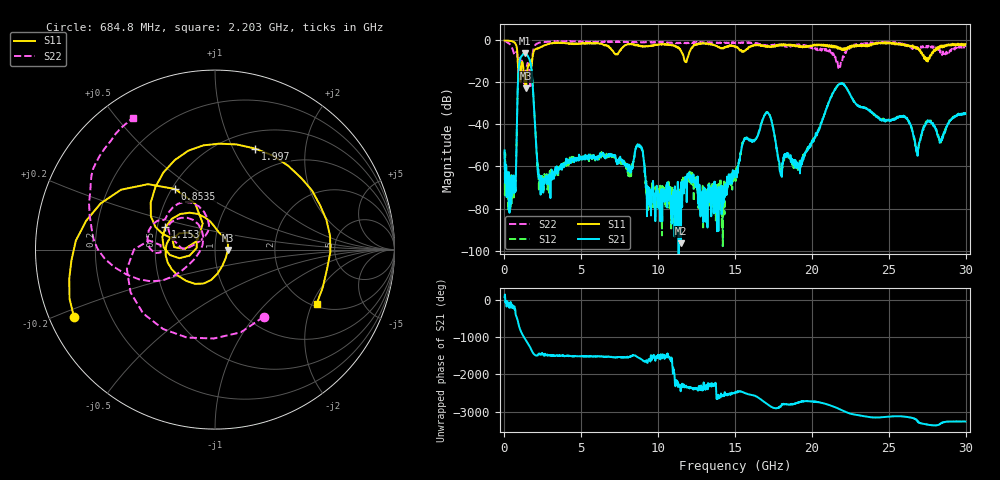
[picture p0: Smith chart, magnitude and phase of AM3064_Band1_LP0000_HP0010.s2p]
# Hz S DB R 50.0
!freq dBS11 angS11 dBS21 angS21 dBS12 angS12 dBS22 angS22
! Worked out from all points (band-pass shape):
!   1600 points, 10 MHz to 29.98 GHz, reference 50 ohm
!   highest |S21| = -6.23 dB at 1.322 GHz (marker M1); lowest = -96.5 dB at 11.48 GHz (marker M2)
!   |S21| within 3 dB of the highest: 1.008 GHz to 1.641 GHz (632.8 MHz wide, 47.8 % of centre)
!   lowest |S11| = -22.9 dB at 1.397 GHz (marker M3), VSWR 1.16, Z = 57.7 - j0.151 ohm
!   |S11| at or under -10 dB: 865.7 MHz to 1.796 GHz (930 MHz wide, 69.9 % of centre); 11.74 GHz to 11.85 GHz (101.1 MHz wide, 0.857 % of centre); 27.53057 GHz to 27.5447 GHz (14.13 MHz wide, 0.0513 % of centre)
!   |S22| runs from -22.7 to -0.2 dB; largest |S21 - S12| = 0.0053
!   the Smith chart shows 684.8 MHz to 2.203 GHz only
!   S11 on the Smith chart (normalised r, x): 684.8 MHz: 0.07, -0.22; 853.5 MHz: 0.52, +0.42; 1.153 GHz: 0.55, +0.15; 1.997 GHz: 0.69, +1.23; 2.203 GHz: 2.10, -2.16
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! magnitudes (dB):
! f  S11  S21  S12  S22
! 10 MHz  -0.1  -52.3  -53.0  -0.2
! 684.8 MHz  -1.2  -65.7  -70.7  -6.7
! 853.5 MHz  -7.9  -25.4  -25.3  -8.6
! 1.153 GHz  -10.4  -7.2  -7.1  -10.1
! 1.322 GHz  -20.4  -6.2  -6.2  -19.0
! 1.397 GHz  -22.9  -6.5  -6.4  -14.3
! 1.716 GHz  -12.7  -11.4  -11.4  -18.2
! 1.997 GHz  -4.4  -41.3  -41.1  -2.3
! 2.203 GHz  -3.9  -61.4  -64.0  -1.3
! 5.015 GHz  -1.5  -56.2  -56.1  -0.8
! 8.763 GHz  -2.7  -50.6  -50.3  -1.0
! 9.382 GHz  -2.7  -70.7  -74.8  -0.9
! 10 GHz  -2.0  -72.9  -77.6  -0.9
! 11.48 GHz  -4.9  -96.5  -67.6  -1.2
! 15 GHz  -3.1  -63.5  -64.1  -1.3
! 17.03 GHz  -2.9  -34.3  -34.5  -2.6
! 17.97 GHz  -2.4  -63.6  -62.5  -2.2
! 19.99 GHz  -2.7  -49.0  -48.0  -3.5
! 21.85 GHz  -3.5  -20.6  -20.4  -12.2
! 25 GHz  -1.0  -38.0  -37.8  -1.0
! 26.85 GHz  -4.2  -52.7  -53.9  -3.1
! 29.98 GHz  -1.8  -35.0  -34.8  -3.1
